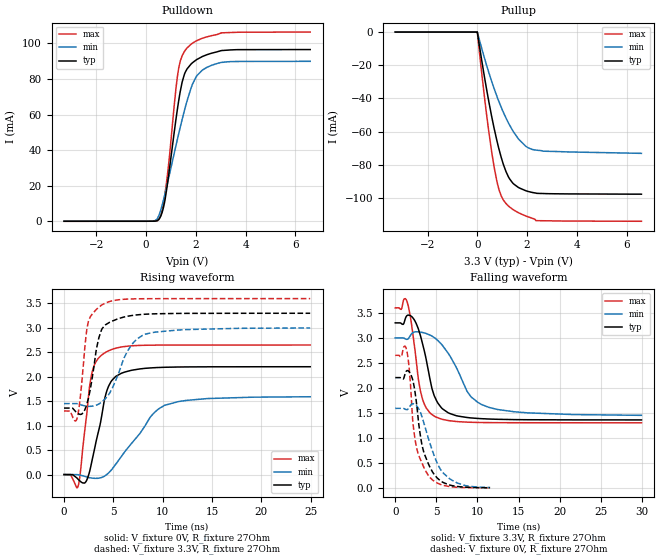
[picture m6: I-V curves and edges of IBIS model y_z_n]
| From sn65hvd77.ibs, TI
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[Model]   y_z_n
Model_type   Output
Polarity   Non-Inverting
Vmeas = 1.65
Vref = 1.956
Cref = 50pF
Rref = 27
|   typ   min   max
|   (nom PVT)   (fast PVT)   (slow PVT)
|Avergae
C_comp   1.500e-11   1.433e-11   1.761e-11
| Where nom  PVT is Nominal Process, 3.3V, 27C
|   Fast PVT is Strong Process,  3.6V, -40C
|   Slow PVT is Weak Process,   3V, 150C
[Voltage Range]   3.3   3   3.6
|Ambient Temperature   25   125   -40
|Junction Temperature
[Temperature Range]   27   150   -40
[Pullup Reference]   3.3   3   3.6
[Pulldown Reference]   0   0   0
[Power Clamp Reference]   3.3   3   3.6
[GND Clamp Reference]   0   0   0
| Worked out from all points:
|   slope of the pulldown table from 0 to 0.495 V, typ, clamps not added: 584 ohm
|   slope of the pullup table from 0 to 0.495 V, typ, clamps not added: 11.1 ohm
|   falling waveform, V_fixture 3.3V, R_fixture 27Ohm: 20-80 % time 1.74ns typ, 3.22ns min, 1.26ns max; typ from 3.3 V to 1.36 V
|   rising waveform, V_fixture 0V, R_fixture 27Ohm: 20-80 % time 1.43ns typ, 3.56ns min, 984ps max; typ from 0 V to 2.21 V
|   rising waveform, V_fixture 3.3V, R_fixture 27Ohm: 20-80 % time 1.05ns typ, 2.12ns min, 744ps max; typ from 1.36 V to 3.3 V
|   falling waveform, V_fixture 0V, R_fixture 27Ohm: 20-80 % time 1.6ns typ, 2.17ns min, 1.33ns max; typ from 2.21 V to 0.005 V
[Pulldown]
|   Voltage   I(typ)   I(min)   I(max)
-3.3V     -6.612uA   -9.318uA   -6.374uA
336mV     41.43uA    229.2uA    18.75uA
519.6mV   1.175mA    3.381mA    1.076mA
670.8mV   6.19mA     10.37mA    7.974mA
847.2mV   19.71mA    20.58mA    24.58mA
1.207V    57.83mA    42.86mA    75.34mA
1.311V    67.7mA     49.13mA    85.95mA
1.541V    82.6mA     62.22mA    95.46mA
1.815V    88.49mA    75.13mA    99.61mA
2.253V    92.56mA    84.88mA    102.8mA
3.021V    95.98mA    89.33mA    105.9mA
6.6V      96.55mA    89.94mA    106.4mA
[Pullup]
|   Voltage   I(typ)   I(min)   I(max)
-3.3V     13.22uA    17.2uA     13.33uA
0V        0A         0A         0A
372mV     -34.39mA   -19.93mA   -49.55mA
672mV     -57.7mA    -33.86mA   -80.94mA
816mV     -67.2mA    -39.81mA   -91.73mA
955.2mV   -75.16mA   -45.09mA   -98.48mA
1.155V    -84.1mA    -51.84mA   -103.3mA
1.296V    -88.39mA   -56mA      -105.3mA
1.68V     -93.83mA   -64.82mA   -109mA
2.212V    -96.61mA   -70.72mA   -112.2mA
2.358V    -97mA      -71.09mA   -113.6mA
6.6V      -97.65mA   -73.05mA   -114mA
[Ramp]
R_load = 27
|   typ   min   max
dV/dt_r   1.32354/1.42664e-09   0.955069/3.54964e-09   1.59029/9.8239e-10
dV/dt_f   1.1635/1.73463e-09   0.928529/3.17417e-09   1.3782/1.25496e-09
[Falling Waveform]
V_fixture = 3.3V
V_fixture_min = 3V
V_fixture_max = 3.6V
R_fixture = 27Ohm
|   Time   V(typ)   V(min)   V(max)
0s        3.3V       3V         3.6V
1.385ns   3.439V     2.971V     3.746V
2.42ns    3.33V      3.12V      2.727V
2.835ns   3.167V     3.12V      2.151V
3.315ns   2.887V     3.107V     1.777V
4.855ns   1.804V     2.992V     1.426V
6.44ns    1.503V     2.693V     1.349V
9.205ns   1.401V     1.823V     1.314V
11.42ns   1.379V     1.61V      1.307V
29.95ns   1.361V     1.452V     1.303V
[Rising Waveform]
V_fixture = 0V
V_fixture_min = 0V
V_fixture_max = 0V
R_fixture = 27Ohm
|   Time   V(typ)   V(min)   V(max)
0s        11.3nV     107.3nV    12.29nV
1.415ns   -92.8mV    -3.105mV   -247.8mV
1.68ns    -143.5mV   -14.08mV   83.14mV
2.22ns    -145.8mV   -43.62mV   1.098V
2.805ns   253.8mV    -71.44mV   2.057V
3.43ns    831.1mV    -76.28mV   2.367V
4.29ns    1.68V      -6.438mV   2.509V
5.805ns   2.072V     368.1mV    2.61V
10.18ns   2.195V     1.415V     2.649V
24.95ns   2.206V     1.592V     2.65V
[Rising Waveform]
V_fixture = 3.3V
V_fixture_min = 3V
V_fixture_max = 3.6V
R_fixture = 27Ohm
|   Time   V(typ)   V(min)   V(max)
0s        1.36V      1.452V     1.301V
1.295ns   1.269V     1.452V     1.131V
1.61ns    1.232V     1.432V     1.511V
2.06ns    1.305V     1.408V     2.485V
2.645ns   1.725V     1.396V     3.222V
3.485ns   2.758V     1.439V     3.417V
4.205ns   3.064V     1.554V     3.51V
6.465ns   3.24V      2.537V     3.59V
8.275ns   3.281V     2.874V     3.597V
24.95ns   3.3V       2.999V     3.6V
[Falling Waveform]
V_fixture = 0V
V_fixture_min = 0V
V_fixture_max = 0V
R_fixture = 27Ohm
|   Time   V(typ)   V(min)   V(max)
0s        2.206V     1.592V     2.652V
1.31ns    2.328V     1.568V     2.799V
1.635ns   2.334V     1.592V     2.491V
2.125ns   2.161V     1.685V     1.352V
2.42ns    1.901V     1.668V     957.4mV
3.245ns   860.7mV    1.427V     502.7mV
4.02ns    487mV      997.5mV    252.2mV
5.13ns    195.8mV    484.8mV    97.31mV
6.545ns   62.87mV    193.8mV    30.64mV
11.54ns   5.336mV    10.73mV    3.634mV
